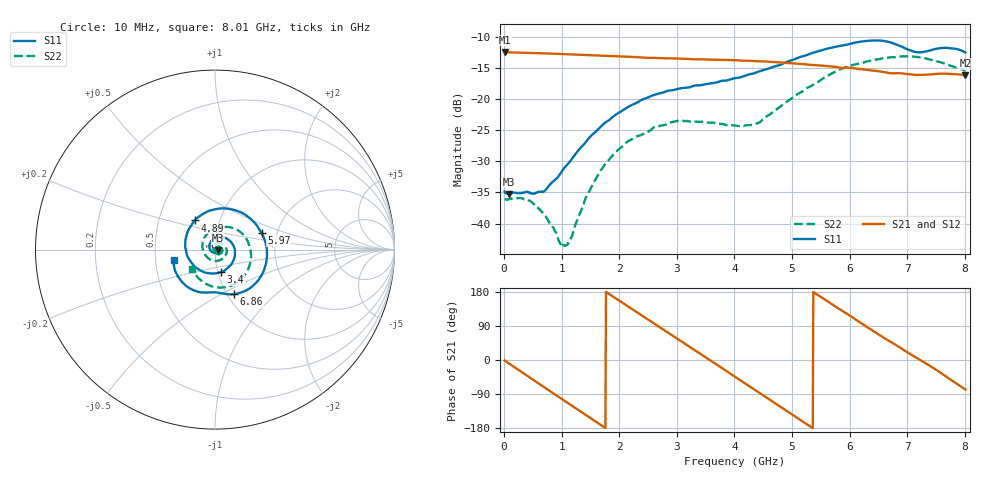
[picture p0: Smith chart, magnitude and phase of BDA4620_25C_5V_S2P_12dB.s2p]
!Agilent Technologies,E5071B,MY42404982,A.09.10
!Date: Wed May 06 09:00:41 2026
!Data & Calibration Information:
!Freq	S11:SOLT2(ON)	S21:SOLT2(ON)	S12:SOLT2(ON)	S22:SOLT2(ON)
# Hz S RI R 50
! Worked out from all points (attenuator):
!   801 points, 10 MHz to 8.01 GHz, reference 50 ohm
!   highest |S21| = -12.43 dB at 10 MHz (marker M1); lowest = -16.2 dB at 8.01 GHz (marker M2)
!   lowest |S11| = -35.2 dB at 80 MHz (marker M3), VSWR 1.04, Z = 51.7 - j0.381 ohm
!   |S11| at or under -10 dB: start of sweep to end of sweep
!   |S22| runs from -43.6 to -13.1 dB; largest |S21 - S12| = 0.0011
!   S11 on the Smith chart (normalised r, x): 10 MHz: 1.04, -0.00; 3.4 GHz: 1.04, -0.26; 4.89 GHz: 0.76, +0.26; 5.97 GHz: 1.66, +0.33; 6.86 GHz: 1.07, -0.57; 8.01 GHz: 0.62, -0.08
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1e7  0.0181 -0.00141  0.239 -0.00514  0.2393 -0.00524  0.0157 -0.000727
8e7  0.017 -0.00368  0.2353 -0.0354  0.2355 -0.0358  0.0156 -0.00118
4.9e8  0.00481 -0.0168  0.1488 -0.1814  0.149 -0.1817  0.0123 -0.00804
7.1e8  -0.00848 -0.0163  0.0677 -0.2231  0.0675 -0.2235  0.00609 -0.00993
1.03e9  -0.0273 -0.000985  -0.0622 -0.2215  -0.0625 -0.2219  -0.00474 -0.00479
1.14e9  -0.0302 0.00806  -0.1036 -0.2045  -0.1039 -0.2047  -0.00728 -0.000914
1.35e9  -0.0299 0.0289  -0.1693 -0.1515  -0.1695 -0.1517  -0.00969 0.00885
1.59e9  -0.0161 0.0523  -0.2143 -0.0681  -0.2145 -0.0682  -0.00684 0.0217
1.9e9  0.0202 0.0698  -0.2155 0.052  -0.2159 0.0521  0.00735 0.0351
2.68e9  0.1108 -0.00354  0.00484 0.2138  0.00508 0.2141  0.0582 0.0164
3.4e9  0.0339 -0.1246  0.1996 0.0613  0.1999 0.0612  0.0445 -0.0483
4.01e9  -0.1129 -0.0942  0.1473 -0.143  0.1475 -0.1433  -0.0281 -0.0547
4.42e9  -0.1657 0.0162  0.0165 -0.2007  0.0163 -0.2011  -0.0644 -0.00675
4.89e9  -0.1128 0.1622  -0.133 -0.1435  -0.1331 -0.144  -0.0513 0.0784
5.35e9  0.0466 0.2298  -0.1883 -0.00424  -0.1885 -0.00431  0.0333 0.1247
5.97e9  0.2592 0.0922  -0.0903 0.1544  -0.0904 0.1547  0.1702 0.0666
6.33e9  0.2843 -0.0766  0.0168 0.1706  0.017 0.1707  0.2008 -0.0238
6.68e9  0.1837 -0.222  0.1027 0.1253  0.1031 0.1256  0.1786 -0.1213
6.86e9  0.1046 -0.2481  0.1337 0.0907  0.134 0.0908  0.1477 -0.1624
7.19e9  0.00065 -0.2376  0.156 0.00894  0.1564 0.00897  0.0585 -0.2096
7.54e9  -0.1129 -0.229  0.139 -0.0795  0.1393 -0.0794  -0.0403 -0.196
8.01e9  -0.2301 -0.057  0.0332 -0.152  0.0336 -0.1524  -0.1302 -0.1075
